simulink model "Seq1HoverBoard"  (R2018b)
settings: Solver=VariableStepAuto  StartTime=0.0  StopTime=5  RelTol=1e-3
libraries: fl_lib x8, nesl_utility x5, elec_lib x1

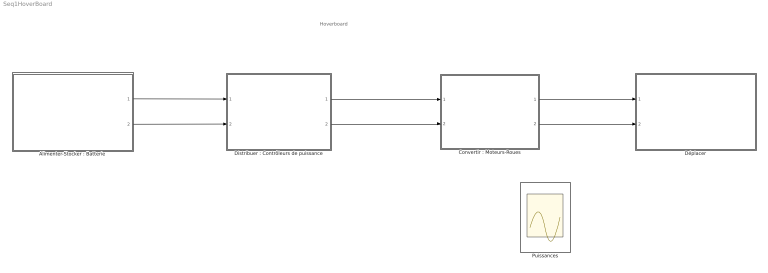
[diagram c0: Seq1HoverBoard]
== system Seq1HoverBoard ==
  note: Hoverboard
  "Alimenter-Stocker : Batterie" : Subsystem  mask{Uchar=0, Ucoup=32, Q=0}
      mask prompts: Uchar "Tension fin charge (V)"; Ucoup "Tension de coupure (V)"; Q "Capacité (en  Ah)"
  "Convertir : Moteurs-Roues" : Subsystem  mask{eta=0.8, R=0}
      mask prompts: eta "eta : rendement"; R "Diamètre de la roue (m)"
  "Distribuer : Contrôleurs de puissance" : Subsystem  mask{R=90}
      mask prompts: R "rendement (%)"
  Déplacer : Subsystem  mask{masseProduit=0, masseConducteur=0, pente=0}
      mask prompts: masseProduit "Masse du produit en kg"; masseConducteur "MAsse du conducteur en kg"; pente "pente en %"
  Puissances : Scope  NumInputPorts=3
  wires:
  ? -> Puissances/1  "Pbatt"
  ? -> Puissances/3  "Proues"
  ? -> Puissances/2  "Pcontroleur"
  "Convertir : Moteurs-Roues"/2(V(m/s)) -> Déplacer/2(In1)
  "Convertir : Moteurs-Roues"/1(Froue) -> Déplacer/1(In2)
  "Alimenter-Stocker : Batterie"/1(Out1) -> "Distribuer : Contrôleurs de puissance"/1(Ue)
  "Alimenter-Stocker : Batterie"/2(Out2) -> "Distribuer : Contrôleurs de puissance"/2(Ie)
  "Distribuer : Contrôleurs de puissance"/1(Us) -> "Convertir : Moteurs-Roues"/1(In1)
  "Distribuer : Contrôleurs de puissance"/2(Is) -> "Convertir : Moteurs-Roues"/2(Idistrib)

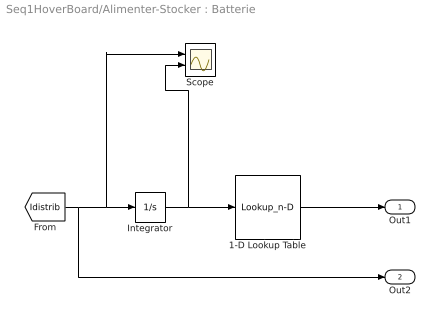
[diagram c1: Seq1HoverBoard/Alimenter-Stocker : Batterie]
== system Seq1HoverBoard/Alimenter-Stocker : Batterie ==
  1-D Lookup Table : Lookup_n-D  NumberOfTableDimensions=1  BreakpointsForDimension1=[0;Q*3600]  Table=[Uchar;Ucoup]  InternalRulePriority=Speed  RndMeth=Simplest
  Integrator : Integrator
  Scope : Scope  NumInputPorts=2
  Out1 : Outport
  Out2 : Outport  Port=2
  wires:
  1-D Lookup Table/1 -> Out1/1
  [Idistrib] -> Out2/1, Scope/1, Integrator/1
  Integrator/1 -> Scope/2, 1-D Lookup Table/1

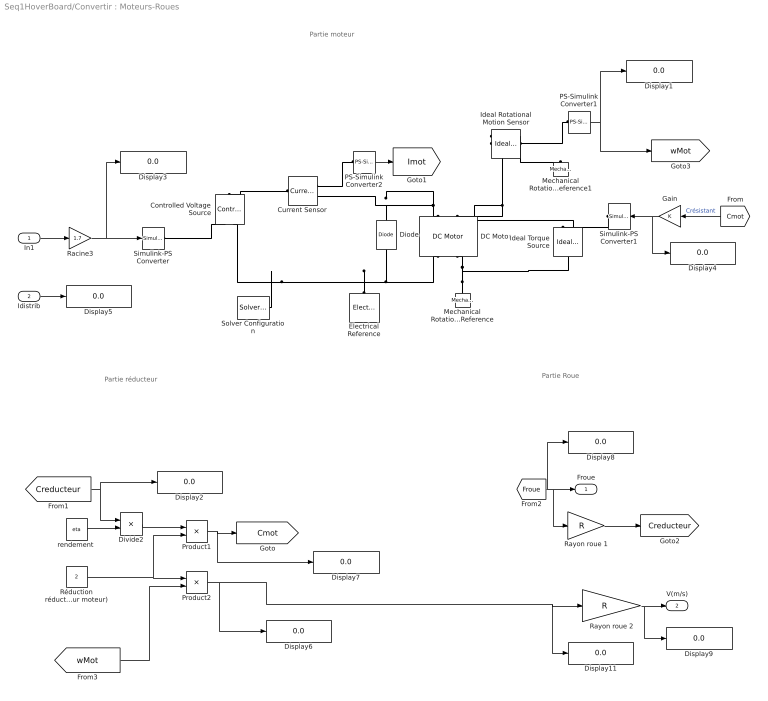
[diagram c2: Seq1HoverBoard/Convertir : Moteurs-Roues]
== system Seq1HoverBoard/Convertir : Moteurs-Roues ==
  note: Partie moteur
  note: Partie Roue
  note: Partie réducteur
  In1 : Inport
  Idistrib : Inport  Port=2
  Controlled Voltage Source : fl_lib/Electrical/Electrical Sources/Controlled Voltage Source
  Current Sensor : fl_lib/Electrical/Electrical Sensors/Current Sensor
  DC Motor : elec_lib/Actuators & Drivers/Rotational Actuators/DC Motor  parameterization=2  Ra=0.35 Ohm  La=5.61e-3 mH  emf_or_torque=1  Kv=0.1 V/(rad/s)  Ki=0.105 N*m/A  T_stall=35 N*m  w_max=65 rpm  w_rated=2000 rpm  P_rated=1000 W  V_rated=36 V  J=340 g*cm^2  lam_param=2  lam=1e-8 N*m/(rad/s)  i_noload=2.96 A  V_i_noload=36 V  speed0=0 rpm  alpha=0.00393 1/K  Tmeas=25 C  thermal_mass=100 J/K  initial_temperature=25 C
  Diode : fl_lib/Electrical/Electrical Elements/Diode  Vf=0.6 V  Ron=0.3 Ohm  Goff=1e-8 1/Ohm  i_specify=off  i_priority=None  i=0 A  i_nominal_specify=off  i_nominal_unit=A  i_nominal_value=1  v_specify=off  v_priority=None  v=0 V  v_nominal_specify=off  v_nominal_unit=V  v_nominal_value=1
  Display{1..9,11} (10 alike) : Display
  Divide2 : Product  Inputs=*/
  Electrical Reference : fl_lib/Electrical/Electrical Elements/Electrical Reference
  Gain : Gain
  Ideal Rotational Motion Sensor : fl_lib/Mechanical/Mechanical Sensors/Ideal Rotational Motion Sensor  offset=0 rad
  Ideal Torque Source : fl_lib/Mechanical/Mechanical Sources/Ideal Torque Source
  Mechanical Rotational Reference : fl_lib/Mechanical/Rotational Elements/Mechanical Rotational Reference
  Mechanical Rotational Reference1 : fl_lib/Mechanical/Rotational Elements/Mechanical Rotational Reference
  PS-Simulink Converter1 : nesl_utility/PS-Simulink Converter  PhysicalDomain=network_engine_domain  SubClassName=ps_output  LeftPortType=input  RightPortType=output  PseudoPeriodic=off  Frequencies=[]  Unit=rad/s  AffineConversion=off
  PS-Simulink Converter2 : nesl_utility/PS-Simulink Converter  PhysicalDomain=network_engine_domain  SubClassName=ps_output  LeftPortType=input  RightPortType=output  PseudoPeriodic=off  Frequencies=[]  Unit=1  AffineConversion=off
  Product1 : Product
  Product2 : Product  Inputs=**
  Racine3 : Gain  Gain=1.7
  Rayon roue 1 : Gain  Gain=R
  Rayon roue 2 : Gain  Gain=R
  Réduction réducteur (compense erreur moteur) : Constant  Value=2
  Simulink-PS Converter : nesl_utility/Simulink-PS Converter  PhysicalDomain=network_engine_domain  SubClassName=ps_input  LeftPortType=input  RightPortType=output  PseudoPeriodic=off  Frequencies=[]  NoiseDistribution=none  NoiseParameters=[]  Unit=1  AffineConversion=off  FilteringAndDerivatives=provide  SimscapeFilterOrder=1  InputFilterTimeConstant=0.001  UdotUserProvided=0
  Simulink-PS Converter1 : nesl_utility/Simulink-PS Converter  PhysicalDomain=network_engine_domain  SubClassName=ps_input  LeftPortType=input  RightPortType=output  PseudoPeriodic=off  Frequencies=[]  NoiseDistribution=none  NoiseParameters=[]  Unit=1  AffineConversion=off  FilteringAndDerivatives=zero  SimscapeFilterOrder=1  InputFilterTimeConstant=.001  UdotUserProvided=0
  Solver Configuration : nesl_utility/Solver Configuration  PhysicalDomain=network_engine_domain  SubClassName=solver  LeftPortType=input  RightPortType=generic  Tones=[]  Harmonics=[]  SimulateNoise=off  Profile=off  UseLocalSampling=off  EnableSwitchedLinearOptims=on  FrequencyDomain=off  UseCCode=off  RelTol=0.001  AbsTol=1e-06  MinStep=1e-09  ToWorkspace=off  RevertToSquareIcSolve=off  NumHomotopyIterations=100  PhasorMode=off  PhasorModeNumHarmonics=1  DoDC=off  ResidualTolerance=1e-9  UseLocalSolver=on  LocalSolverChoice=NE_BACKWARD_EULER_ADVANCER  LocalSolverSampleTime=.001  DoFixedCost=on  MaxNonlinIter=3  MaxModeIter=2  LinearAlgebra=Sparse  EquationFormulation=NE_TIME_EF  DelaysMemoryBudget=1024  AutomaticFiltering=on  FilteringTimeConstant=0.001  PartitionStorageMethod=AS_NEEDED  PartitionMemoryBudget=1024
  "rendement " : Constant  Value=eta  VectorParams1D=off
  Froue : Outport
  V(m/s) : Outport  Port=2
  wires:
  In1/1 -> Racine3/1
  PS-Simulink Converter2/1 -> [Imot]
  [Cmot] -> Gain/1  "Crésistant"
  PS-Simulink Converter1/1 -> [wMot], Display1/1
  Gain/1 -> Simulink-PS Converter1/1, Display4/1
  Racine3/1 -> Simulink-PS Converter/1, Display3/1
  Divide2/1 -> Product1/1
  [Creducteur] -> Display2/1, Divide2/1
  Réduction réducteur (compense erreur moteur)/1 -> Product2/1, Product1/2
  Product1/1 -> Display7/1, [Cmot]
  "rendement "/1 -> Divide2/2
  [wMot] -> Product2/2
  Product2/1 -> Display6/1, Display11/1, Rayon roue 2/1
  Rayon roue 1/1 -> [Creducteur]
  [Froue] -> Display8/1, Rayon roue 1/1, Froue/1
  Rayon roue 2/1 -> Display9/1, V(m/s)/1
  Idistrib/1 -> Display5/1
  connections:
  Ideal Rotational Motion Sensor/RConn1 -- Mechanical Rotational Reference1/LConn1
  PS-Simulink Converter1/LConn1 -- Ideal Rotational Motion Sensor/RConn2
  DC Motor/LConn1 -- Diode/RConn1 -- Current Sensor/RConn2
  DC Motor/RConn2 -- Ideal Torque Source/LConn1 -- Mechanical Rotational Reference/LConn1
  Electrical Reference/LConn1 -- Diode/LConn1 -- DC Motor/RConn1 -- Solver Configuration/RConn1 -- Controlled Voltage Source/RConn2
  Ideal Rotational Motion Sensor/LConn1 -- Ideal Torque Source/RConn2 -- DC Motor/LConn2
  Simulink-PS Converter/RConn1 -- Controlled Voltage Source/RConn1
  Current Sensor/LConn1 -- Controlled Voltage Source/LConn1
  PS-Simulink Converter2/LConn1 -- Current Sensor/RConn1
  Simulink-PS Converter1/RConn1 -- Ideal Torque Source/RConn1

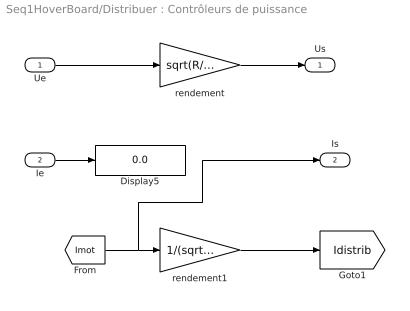
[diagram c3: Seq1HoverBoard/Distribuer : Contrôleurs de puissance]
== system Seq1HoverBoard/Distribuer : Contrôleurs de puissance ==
  Ue : Inport
  Ie : Inport  Port=2
  Display5 : Display
  rendement : Gain  Gain=sqrt(R/100)
  rendement1 : Gain  Gain=1/(sqrt(R/100))
  Us : Outport
  Is : Outport  Port=2
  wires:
  Ue/1 -> rendement/1
  rendement/1 -> Us/1
  Ie/1 -> Display5/1
  [Imot] -> Is/1, rendement1/1
  rendement1/1 -> [Idistrib]

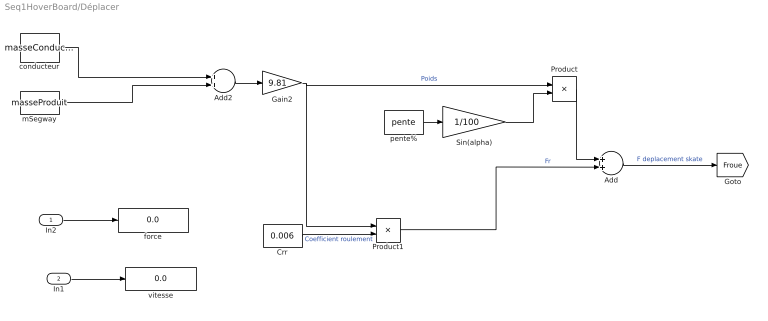
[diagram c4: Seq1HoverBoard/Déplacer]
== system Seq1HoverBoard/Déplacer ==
  In2 : Inport
  In1 : Inport  Port=2
  Add : Sum
  Add2 : Sum
  Crr : Constant  Value=0.006
  Gain2 : Gain  Gain=9.81
  Product : Product
  Product1 : Product
  Sin(alpha) : Gain  Gain=1/100
  conducteur : Constant  Value=masseConducteur
  force : Display
  mSegway : Constant  Value=masseProduit
  pente% : Constant  Value=pente
  vitesse : Display
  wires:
  Add/1 -> [Froue]  "F deplacement skate"
  Gain2/1 -> Product/1, Product1/1  "Poids"
  Product/1 -> Add/1
  pente%/1 -> Sin(alpha)/1
  Crr/1 -> Product1/2  "Coefficient roulement"
  conducteur/1 -> Add2/1
  Add2/1 -> Gain2/1
  mSegway/1 -> Add2/2
  In1/1 -> vitesse/1
  In2/1 -> force/1
  Sin(alpha)/1 -> Product/2
  Product1/1 -> Add/2  "Fr"
